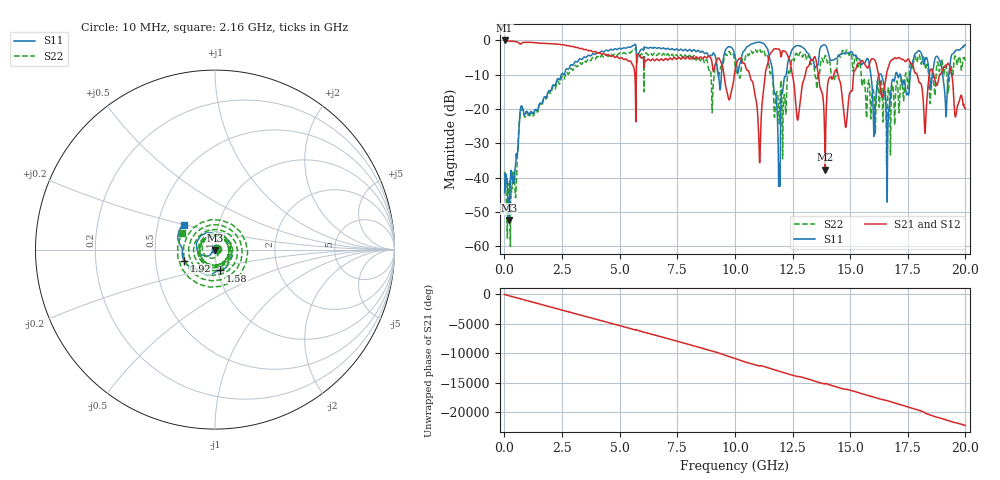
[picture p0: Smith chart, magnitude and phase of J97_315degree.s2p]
!Keysight Technologies,N5222A,MY51421036,A.10.65.16
!Date: Friday, March 31, 2023 15:14:03
!Correction: S11(Full 2 Port(1,2))
!S21(Full 2 Port(1,2))
!S12(Full 2 Port(1,2))
!S22(Full 2 Port(1,2))
!S2P File: Measurements: S11, S21, S12, S22:
# Hz S  dB  R 50
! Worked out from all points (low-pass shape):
!   2000 points, 10 MHz to 20 GHz, reference 50 ohm
!   highest |S21| = -0.02 dB at 10 MHz (marker M1); lowest = -37.7 dB at 13.92 GHz (marker M2)
!   |S21| within 3 dB of the highest: start of sweep to 3.637 GHz; 11.64 GHz to 11.96 GHz (319.8 MHz wide, 2.71 % of centre)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
!   lowest |S11| = -52.5 dB at 200 MHz (marker M3), VSWR 1.00, Z = 49.9 - j0.226 ohm
!   |S11| at or under -10 dB: start of sweep to 2.467 GHz; 11.64 GHz to 12.23 GHz (584 MHz wide, 4.89 % of centre); 16.35 GHz to 16.97 GHz (616.7 MHz wide, 3.7 % of centre)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
!   |S22| runs from -60.0 to -2.1 dB; largest |S21 - S12| = 0.01
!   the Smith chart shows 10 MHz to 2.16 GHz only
!   S11 on the Smith chart (normalised r, x): 10 MHz: 1.01, +0.01; 1.58 GHz: 1.03, -0.24; 1.92 GHz: 0.70, -0.09; 2.16 GHz: 0.68, +0.20
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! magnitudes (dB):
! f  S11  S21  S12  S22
! 10 MHz  -44.4  0.0  -0.1  -38.3
! 200 MHz  -52.5  -0.2  -0.2  -41.8
! 730 MHz  -19.2  -0.9  -0.9  -20.5
! 1.58 GHz  -18.5  -0.8  -0.8  -18.4
! 1.92 GHz  -14.8  -0.9  -0.9  -15.0
! 2.16 GHz  -13.1  -1.0  -1.0  -13.7
! 3.35 GHz  -5.6  -2.4  -2.3  -7.0
! 6.68 GHz  -2.1  -5.8  -5.8  -3.9
! 10.01 GHz  -4.7  -8.5  -8.5  -7.6
! 11.07 GHz  -0.5  -35.7  -35.6  -2.6
! 11.54 GHz  -6.1  -3.7  -3.7  -9.8
! 11.9 GHz  -42.6  -2.5  -2.5  -20.1
! 12.42 GHz  -3.9  -7.1  -7.1  -7.7
! 12.74 GHz  -1.5  -23.0  -23.0  -4.8
! 13.34 GHz  -5.7  -5.6  -5.6  -6.1
! 13.92 GHz  -1.4  -37.7  -37.7  -4.4
! 14.36 GHz  -5.4  -8.8  -8.8  -10.5
! 16.67 GHz  -20.6  -7.5  -7.5  -13.7
! 17.89 GHz  -3.5  -9.7  -9.7  -6.4
! 18.25 GHz  -5.6  -27.1  -27.1  -7.6
! 19.15 GHz  -21.3  -7.8  -7.8  -7.2
! 20 GHz  -1.3  -20.0  -20.0  -6.6
